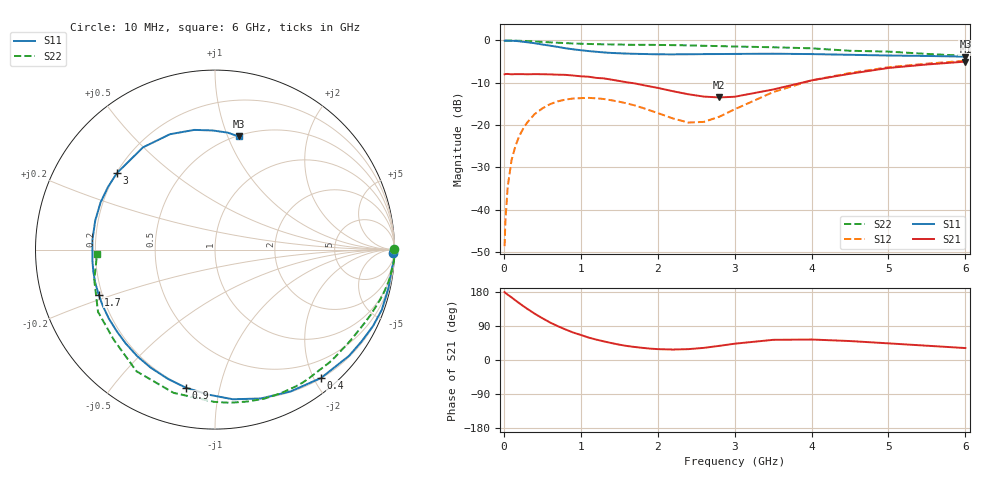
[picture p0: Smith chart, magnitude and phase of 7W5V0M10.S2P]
! Infineon Technologies  Discrete & RF Semiconductors
! BFS17W
! Si NPN RF Bipolar Junction Transistor in SOT323
! VCE = 5 V  IC = 0.1 mA
! Common Emitter S-Parameters:  August  1999
# GHz  S  MA  R  50
!  f  S11  S21  S12  S22
! GHz  MAG  ANG  MAG  ANG  MAG  ANG  MAG  ANG
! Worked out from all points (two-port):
!   36 points, 10 MHz to 6 GHz, reference 50 ohm
!   highest |S21| = -5.01 dB at 6 GHz (marker M1); lowest = -13.5 dB at 2.8 GHz (marker M2)
!   |S21| within 3 dB of the highest: start of sweep to 556.7 MHz; 4.458 GHz to end of sweep
!   lowest |S11| = -3.8 dB at 6 GHz (marker M3), VSWR 4.62, Z = 25.4 + j54.8 ohm
!   |S11| at or under -10 dB: nowhere
!   |S22| runs from -3.6 to 0.0 dB; largest |S21 - S12| = 0.4
!   S11 on the Smith chart (normalised r, x): 10 MHz: 24, -89; 400 MHz: 0.21, -2.11; 900 MHz: 0.20, -0.79; 1.7 GHz: 0.19, -0.18; 3 GHz: 0.20, +0.33; 6 GHz: 0.51, +1.10
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0.01  0.9945 -1.2  0.398 179.3  0.0037 89.4  0.9999 0.1
0.02  0.9999 -2.9  0.401 177.1  0.0072 86.8  0.9851 -0.5
0.05  0.9906 -6.5  0.402 172.4  0.0186 87.7  0.9984 -1.8
0.1  0.9899 -12.6  0.398 165.3  0.0385 82.5  0.9993 -3.6
0.2  0.9778 -25.8  0.4 150.0  0.0741 73.7  0.9909 -7.1
0.4  0.9276 -50.4  0.4 122.3  0.1347 58.0  0.9722 -13.8
0.6  0.8679 -72.9  0.397 99.0  0.1765 44.8  0.95 -19.8
0.9  0.7863 -101.9  0.385 72.6  0.2059 29.1  0.9214 -28.3
1.1  0.7491 -118.6  0.373 59.3  0.2096 21.0  0.9092 -33.7
1.4  0.7118 -140.2  0.344 44.6  0.1961 12.0  0.8979 -41.9
1.7  0.6951 -158.9  0.311 34.4  0.1707 7.6  0.8874 -50.7
2.2  0.6851 175.4  0.251 27.6  0.1195 16.0  0.8802 -65.6
2.4  0.6866 166.4  0.231 28.7  0.107 28.5  0.8748 -71.9
2.6  0.6896 157.6  0.217 32.0  0.109 44.2  0.865 -78.2
2.8  0.6909 149.7  0.212 37.3  0.1253 57.2  0.8574 -84.5
3  0.693 142.1  0.216 43.0  0.1534 65.3  0.8483 -90.3
3.5  0.6968 125.2  0.263 53.2  0.2451 69.6  0.8308 -106.1
4  0.6901 111.3  0.337 54.1  0.3379 63.8  0.8068 -122.8
4.5  0.6768 99.8  0.404 50.0  0.4124 55.8  0.7551 -138.4
5  0.6639 91.1  0.473 43.9  0.4827 48.0  0.7382 -152.0
5.5  0.6555 83.8  0.52 37.7  0.5321 40.4  0.6935 -165.9
6  0.6442 78.2  0.562 31.5  0.5749 33.5  0.6574 -177.9
